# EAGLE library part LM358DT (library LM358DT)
LM358DT, Dual Operational Amplifier 1.1MHz 5 to 28V, 8-Pin SO Source: Datasheet
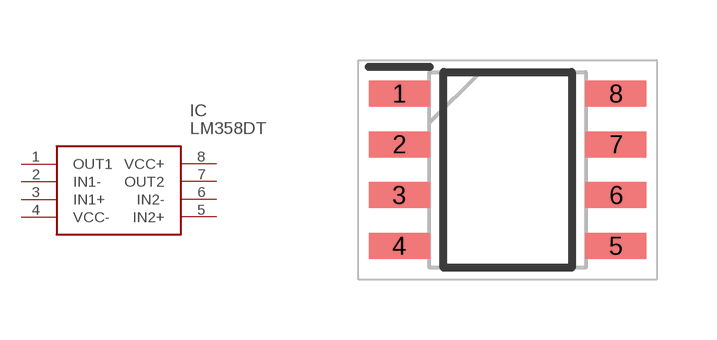
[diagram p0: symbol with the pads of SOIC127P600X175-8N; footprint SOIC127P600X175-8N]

Designator prefix IC

## LM358DT (Arrow_Part_Number: LM358DT; Arrow_Price-Stock: https://www.arrow.com/en/products/lm358dt/stmicroelectronics?region=nac; Description: LM358DT, Dual Operational Amplifier 1.1MHz 5 to 28V, 8-Pin SO; Height: 1.75mm; Manufacturer_Name: STMicroelectronics; Manufacturer_Part_Number: LM358DT; Mouser_Part_Number: 511-LM358DT; Mouser_Price-Stock: https://www.mouser.co.uk/ProductDetail/STMicroelectronics/LM358DT?qs=omvQGv%252BAfzDWfqgV6a5v9A%3D%3D)  [SOIC127P600X175-8N]
1  OUT1
2  IN1-
3  IN1+
4  VCC-
5  IN2+
6  IN2-
7  OUT2
8  VCC+

## Footprint SOIC127P600X175-8N (pad centres in mm)
SO 8_
smd 1.525 x 0.65: 1 -2.712,1.905; 2 -2.712,0.635; 3 -2.712,-0.635; 4 -2.712,-1.905; 5 2.712,-1.905; 6 2.712,-0.635; 7 2.712,0.635; 8 2.712,1.905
